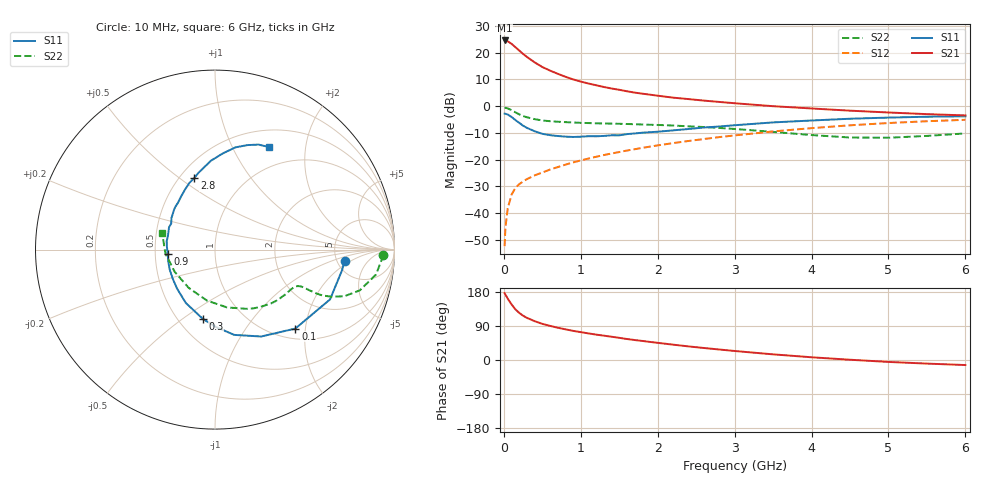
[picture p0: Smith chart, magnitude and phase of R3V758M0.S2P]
! SIEMENS Small Signal Semiconductors
! BFR181
! Si NPN RF Bipolar Junction Transistor in SOT23
! VCE = 0.75 V  IC = 8 mA
! Common Emitter S-Parameters:  May  1996
# GHz  S  MA  R  50
!  f  S11  S21  S12  S22
! GHz  MAG  ANG  MAG  ANG  MAG  ANG  MAG  ANG
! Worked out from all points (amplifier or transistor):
!   36 points, 10 MHz to 6 GHz, reference 50 ohm
!   highest |S21| = 24.6 dB at 10 MHz (marker M1)
!   |S21| within 3 dB of that: start of sweep to 169.6 MHz
!   unconditionally stable (mu >= 1): 435.1 MHz to end of sweep
!   at 250 MHz: K = 0.73, MSG = 23.9 dB, |S12| = -28.2 dB
!   at 1.4 GHz: K = 1.30, MAG = 8.9 dB, |S12| = -17.7 dB
!   at 6 GHz: K = 1.04, MAG = -0.4 dB, |S12| = -5.1 dB
!   S11 on the Smith chart (normalised r, x): 10 MHz: 5.85, -1.52; 100 MHz: 1.22, -1.76; 300 MHz: 0.66, -0.60; 900 MHz: 0.58, -0.03; 2.8 GHz: 0.59, +0.57; 6 GHz: 0.71, +1.40
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0.01  0.7243 -4.9  16.91 176.5  0.0024 88.9  0.9354 -1.8
0.02  0.7173 -9.2  16.68 172.7  0.0052 80.4  0.9299 -3.6
0.05  0.6985 -23.4  16.3 162.1  0.0121 78.9  0.9078 -8.8
0.1  0.6276 -44.5  14.65 146.7  0.0221 70.6  0.8384 -15.7
0.15  0.5484 -62.0  12.67 133.7  0.0295 63.4  0.7666 -19.8
0.2  0.4871 -77.3  10.97 124.3  0.0347 60.9  0.701 -22.0
0.25  0.4307 -89.4  9.474 116.9  0.0389 58.7  0.6516 -23.1
0.3  0.3918 -100.0  8.317 111.2  0.0431 58.7  0.6188 -23.4
0.4  0.3388 -118.7  6.588 102.5  0.0506 59.2  0.5704 -23.3
0.5  0.3031 -134.2  5.391 95.4  0.0573 60.3  0.5394 -23.1
0.6  0.2863 -145.2  4.623 90.1  0.065 61.1  0.522 -23.2
0.7  0.2759 -156.2  4.028 85.2  0.0723 62.2  0.5104 -23.5
0.9  0.2648 -174.4  3.161 76.9  0.0885 63.8  0.494 -24.6
1.1  0.2733 170.3  2.648 70.2  0.1045 64.8  0.4818 -26.7
1.3  0.2769 159.7  2.28 64.2  0.1215 64.8  0.4735 -29.0
1.6  0.2992 144.3  1.896 55.4  0.1475 64.2  0.4631 -33.2
2.2  0.3519 122.4  1.44 40.5  0.2031 61.1  0.4333 -43.7
2.8  0.4158 106.1  1.198 27.7  0.2634 56.3  0.3906 -57.0
3.5  0.4958 92.6  0.997 14.9  0.336 48.9  0.3293 -78.2
4.5  0.5809 78.7  0.822 0.7  0.4376 35.8  0.2585 -124.8
5.5  0.6332 67.5  0.708 -9.5  0.5218 21.7  0.2771 -175.4
6  0.6456 62.3  0.67 -13.3  0.5546 14.2  0.3087 162.5
